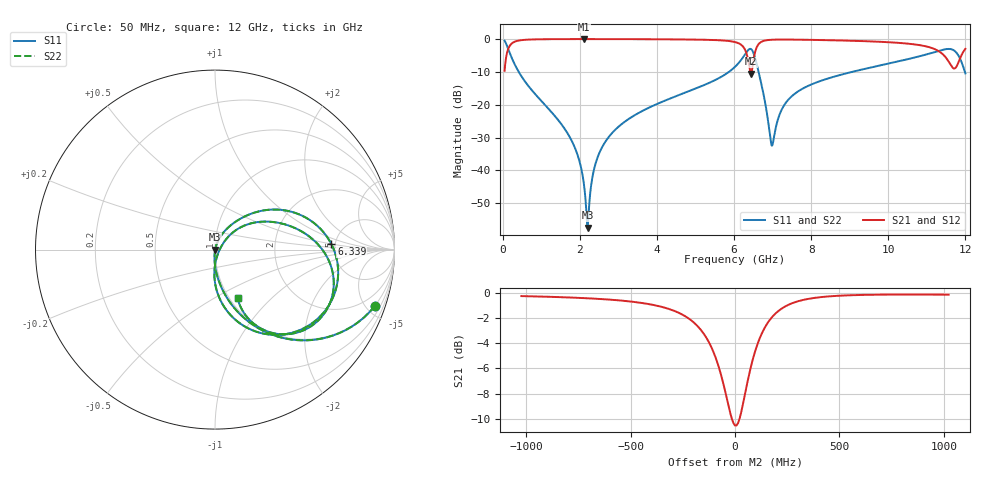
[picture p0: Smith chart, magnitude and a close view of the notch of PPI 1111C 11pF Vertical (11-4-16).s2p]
# GHz S MA R 50
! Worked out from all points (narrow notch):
!   1601 points, 50 MHz to 12 GHz, reference 50 ohm
!   highest |S21| = -0.01 dB at 2.104 GHz (marker M1); lowest = -10.5 dB at 6.436 GHz (marker M2)
!   notch at M2: 10.3 dB deep, 171 MHz wide at half that depth
!   lowest |S11| = -57.4 dB at 2.201 GHz (marker M3), VSWR 1.00, Z = 50.1 - j0.0256 ohm
!   |S11| at or under -10 dB: 416.3 MHz to 5.867 GHz (5.451 GHz wide, 173 % of centre); 6.637 GHz to 9.062 GHz (2.425 GHz wide, 30.9 % of centre); 11.98781 GHz to end of sweep
!   |S22| runs from -57.4 to -0.5 dB; largest |S21 - S12| = 0
!   S11 on the Smith chart (normalised r, x): 50 MHz: 0.98, -5.68; 6.339 GHz: 4.64, +0.49; 12 GHz: 1.09, -0.65
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0.05  0.9444 -19.4  0.3287 70.6  0.3287 70.6  0.9444 -19.4
0.22925  0.527 -59.2  0.8494 30.7  0.8494 30.7  0.527 -59.2
0.4458437  0.2958 -74.8  0.9546 15.1  0.9546 15.1  0.2958 -74.8
1.648313  0.03956 -93.8  0.998 -5.5  0.998 -5.5  0.03956 -93.8
2.044156  0.01026 -91.8  0.9985 -9.1  0.9985 -9.1  0.01026 -91.8
2.103906  0.006372 -87.7  0.9985 -9.6  0.9985 -9.6  0.006372 -87.7
2.201  0.001346 -10.9  0.9985 -10.4  0.9985 -10.4  0.001346 -10.9
2.387719  0.0115 71.0  0.9984 -11.9  0.9984 -11.9  0.0115 71.0
2.664062  0.02744 72.7  0.998 -14.1  0.998 -14.1  0.02744 72.7
4.038312  0.1049 63.9  0.9921 -24.9  0.9921 -24.9  0.1049 63.9
6.025  0.3775 36.1  0.9 -50.0  0.9 -50.0  0.3775 36.1
6.338687  0.6491 2.7  0.5648 -66.6  0.5648 -66.6  0.6491 2.7
6.435781  0.7062 -26.2  0.2976 -37.7  0.2976 -37.7  0.7062 -26.2
6.525406  0.5637 -57.1  0.5603 -2.7  0.5603 -2.7  0.5637 -57.1
6.644906  0.3022 -82.5  0.8475 -14.2  0.8475 -14.2  0.3022 -82.5
6.981  0.02386 -25.4  0.9759 -32.2  0.9759 -32.2  0.02386 -25.4
7.3395  0.1064 44.1  0.9824 -39.6  0.9824 -39.6  0.1064 44.1
8.019156  0.2052 39.8  0.9714 -48.3  0.9714 -48.3  0.2052 39.8
10.01331  0.4245 18.8  0.8943 -69.8  0.8943 -69.8  0.4245 18.8
11.46972  0.6972 -19.0  0.5429 -92.3  0.5429 -92.3  0.6972 -19.0
11.72366  0.6579 -44.1  0.3565 -64.7  0.3565 -64.7  0.6579 -44.1
12  0.2999 -65.2  0.7102 -47.0  0.7102 -47.0  0.2999 -65.2
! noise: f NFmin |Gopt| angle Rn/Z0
0.05  0.0003797  0.8734  1.81  0.0006466
1.372  0.003754  0.674  6.791  0.002212
2.701  0.006305  0.6305  12.55  0.003167
4.031  0.00916  0.6263  18.2  0.00448
5.36  0.01625  0.7104  24.13  0.01058
6.682  0.07563  0.9148  30.77  0.1819
8.012  0.02249  0.702  35.64  0.01344
9.341  0.02513  0.6988  40.53  0.01442
10.67  0.04859  0.8152  46.48  0.04649
12  0.1943  0.9458  52.36  0.6468
